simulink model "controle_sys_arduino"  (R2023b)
settings: Solver=FixedStepAuto  StartTime=0.0  StopTime=inf  RelTol=1e-3  EnableMultiTasking=on
libraries: arduinolib x5

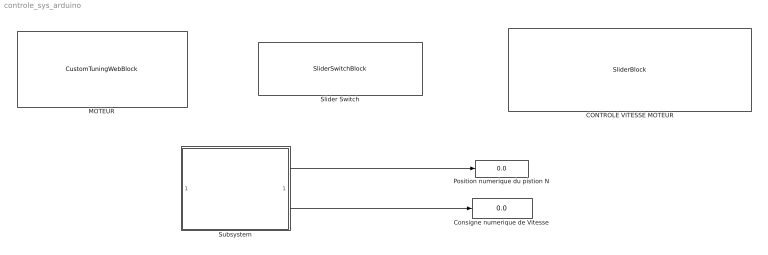
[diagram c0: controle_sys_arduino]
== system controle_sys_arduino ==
  CONTROLE VITESSE MOTEUR : SliderBlock  ScaleMax=255
  Consigne numerique de Vitesse : Display
  MOTEUR : CustomTuningWebBlock  LabelPosition=Hide  ShowInitialText=on  Configuration="{\"components\":[{\"name\":\"CustomSwitchStateComponent\",\"settings\":{\"position\":[0,0,1,1],\"states\":[{\"HitRegion\":{\"position\":[0,0,0.5,1]},\"Image\":{\"position\":[0.13,0,1,0.75],\"size\":[1,0.75],\"src\":\"data:image\\/svg+xml;base64,PHN2ZyB4bWxucz0iaHR0cDovL3d3dy53My5vcmcvMjAwMC9zdmciIHhtbG5zOnhsaW5rPSJodHRwOi8vd3d3LnczLm9yZy8xOTk5L3hsaW5rIiB2aWV3Qm94PSIwIDAgNzUgMjQuOCI+PGRlZnM+PHN0eWxlPi5jbHMtMXtmaWxsOnVybCgjc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"
  Position numerique du pistion N : Display
  Slider Switch : SliderSwitchBlock
  Subsystem : Subsystem
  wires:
  Subsystem/1(Out1) -> Position numerique du pistion N/1
  Subsystem/2(Out2) -> Consigne numerique de Vitesse/1

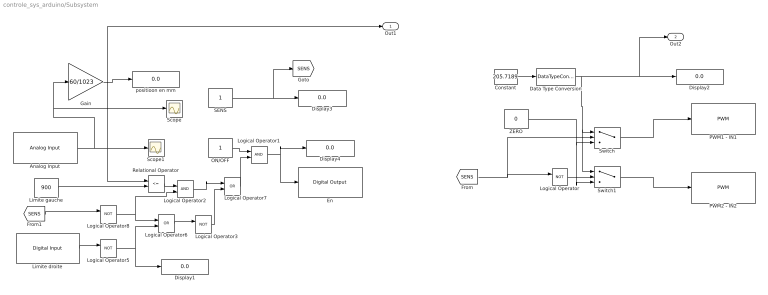
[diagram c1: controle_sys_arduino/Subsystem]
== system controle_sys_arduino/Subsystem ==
  Analog Input : arduinolib/Analog Input  pinNumber=0  ReadResultsOnly=off  ConversionTriggerSource=Software  ExternalTriggerType=uint32( 0 )  OutputDataType=uint16  EnableConversionCompleteNotify=off  EnableOuputStatus=off  SampleTime=-1  blockPlatform=arduino
  Constant : Constant  Value=205.7189
  Data Type Conversion : DataTypeConversion  OutDataTypeStr=uint8
  Display{1..4} (4 alike) : Display
  En : arduinolib/Digital Output  pinNumber=23  Direction=output  blockPlatform=arduino
  Gain : Gain  Gain=60/1023
  Limite droite : arduinolib/Digital Input  pinNumber=25  mode=Input Pullup  Direction=input  SampleTime=0.1  blockPlatform=arduino
  Limite gauche : Constant  Value=900
  Logical Operator{,3,5,8} (4 alike) : Logic  Operator=NOT  AllPortsSameDT=off  OutDataTypeStr=boolean
  Logical Operator1 : Logic  AllPortsSameDT=off  OutDataTypeStr=boolean
  Logical Operator2 : Logic  AllPortsSameDT=off  OutDataTypeStr=boolean
  Logical Operator6 : Logic  Operator=OR  AllPortsSameDT=off  OutDataTypeStr=boolean
  Logical Operator7 : Logic  Operator=OR  AllPortsSameDT=off  OutDataTypeStr=boolean
  ON/OFF : Constant
  PWM1 - IN1 : arduinolib/PWM  pinNumber=4  frequencyType=Default  desiredFrequency=490.2  achievableFrequency=490.2
  PWM2 - IN2 : arduinolib/PWM  pinNumber=5  frequencyType=Default  desiredFrequency=490.2  achievableFrequency=490.2
  Relational Operator : RelationalOperator  Operator=<=  OutDataTypeStr=boolean  RndMeth=Simplest
  SENS : Constant
  Scope : Scope
  Scope1 : Scope
  Switch : Switch  Criteria=u2 > Threshold
  Switch1 : Switch  Criteria=u2 ~= 0
  ZERO : Constant  Value=0
  positioon en mm : Display
  Out1 : Outport
  Out2 : Outport  Port=2
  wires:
  Data Type Conversion/1 -> Switch1/1, Switch/1, Out2/1, Display2/1
  Analog Input/1 -> Gain/1, Scope/1, Out1/1, Relational Operator/1, Scope1/1
  ZERO/1 -> Switch1/3, Switch/3
  Relational Operator/1 -> Logical Operator2/1
  SENS/1 -> [SENS], Display3/1
  Switch1/1 -> PWM2 - IN2/1
  Logical Operator/1 -> Switch1/2
  Logical Operator5/1 -> Logical Operator6/2, Display1/1
  Limite droite/1 -> Logical Operator5/1
  Logical Operator8/1 -> Logical Operator6/1, Logical Operator2/2
  Constant/1 -> Data Type Conversion/1
  Logical Operator7/1 -> Logical Operator1/2
  [SENS] -> Switch/2, Logical Operator/1
  Logical Operator1/1 -> Display4/1, En/1
  Logical Operator2/1 -> Logical Operator7/1
  Limite gauche/1 -> Relational Operator/2
  ON/OFF/1 -> Logical Operator1/1
  Gain/1 -> positioon en mm/1
  Logical Operator3/1 -> Logical Operator7/2
  Logical Operator6/1 -> Logical Operator3/1
  Switch/1 -> PWM1 - IN1/1
  [SENS] -> Logical Operator8/1
